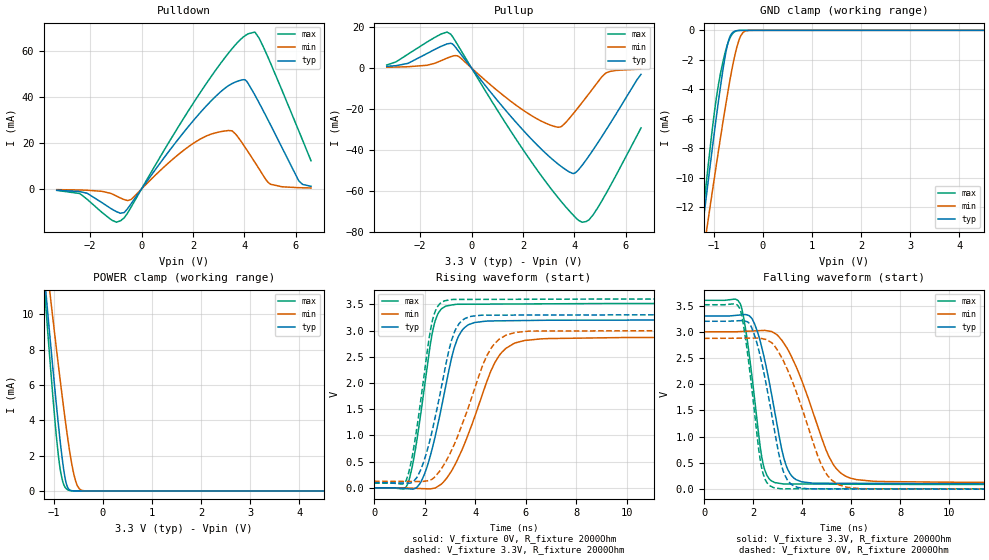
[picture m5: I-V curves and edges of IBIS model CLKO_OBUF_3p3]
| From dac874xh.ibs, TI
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|   CLKO_OBUF_3p3 Model
[Model]   CLKO_OBUF_3p3
Model_type   3-state
Polarity   Non-Inverting
Vmeas = 1.65
Vref = 0
Cref = 2pF
Rref = 100000
|   typ   min   max
C_comp   6.24499E-13   5.18659E-13   6.49121E-13
| Where nom  PVT is Nominal Process, 3.3V, 27C
|   Fast PVT is Strong Process,  3.6V, -40C
|   Slow PVT is Weak Process,   3.0V, 150C
[Voltage Range]   3.3   3   3.6
[Temperature Range]   27   150   -40
[Pullup Reference]   3.3   3   3.6
[Pulldown Reference]   0   -0   0
[Power Clamp Reference]   3.3   3   3.6
[GND Clamp Reference]   0   0   0
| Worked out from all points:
|   slope of the pulldown table from 0 to 0.495 V, typ, clamps not added: 63.8 ohm
|   slope of the pullup table from 0 to 0.495 V, typ, clamps not added: 62.5 ohm
|   GND clamp passes 1 mA (typ) near -0.72 V on its own axis
|   POWER clamp passes 1 mA (typ) near -0.79 V on its own axis
|   falling waveform, V_fixture 3.3V, R_fixture 2000Ohm: 20-80 % time 803ps typ, 1.35ns min, 551ps max; typ from 3.3 V to 0.101 V
|   rising waveform, V_fixture 0V, R_fixture 2000Ohm: 20-80 % time 869ps typ, 1.35ns min, 628ps max; typ from 0 V to 3.2 V
|   rising waveform, V_fixture 3.3V, R_fixture 2000Ohm: 20-80 % time 863ps typ, 1.32ns min, 614ps max; typ from 0.101 V to 3.3 V
|   falling waveform, V_fixture 0V, R_fixture 2000Ohm: 20-80 % time 786ps typ, 1.3ns min, 537ps max; typ from 3.2 V to 0 V
[Pulldown]
|   Voltage   I(typ)   I(min)   I(max)
-3.3V     -518.9uA   -279.8uA   -604.3uA
-2.122V   -1.843mA   -540.5uA   -4.429mA
-815.1mV  -10.56mA   -3.943mA   -13.82mA
-409.2mV  -6.481mA   -4.563mA   -7.949mA
1.591V    23.93mA    16.4mA     29.86mA
2.838V    39.75mA    24.31mA    50.92mA
3.521V    45.83mA    25.31mA    60.97mA
3.957V    47.54mA    19.39mA    66.05mA
4.402V    41.11mA    11.81mA    68.25mA
5.026V    27.83mA    2.052mA    54.68mA
6.125V    3.502mA    572uA      25.23mA
6.6V      1.16mA     444.7uA    12.24mA
[GND Clamp]
|   Voltage   I(typ)   I(min)   I(max)
-3.3V     -72.02mA   -64.29mA   -82.15mA
-1.241V   -13.64mA   -15.69mA   -13.06mA
-1.122V   -10.42mA   -12.98mA   -9.355mA
-993.3mV  -7.012mA   -10.1mA    -5.674mA
-904.2mV  -4.759mA   -8.138mA   -3.641mA
-815.1mV  -2.685mA   -6.23mA    -2.133mA
-726mV    -1.033mA   -4.408mA   -990.6uA
-656.7mV  -325.7uA   -3.092mA   -426.6uA
-577.5mV  -63.94uA   -1.78mA    -100.6uA
-448.8mV  -2.544uA   -357.2uA   -3.784uA
-290.4mV  0A         -7.658uA   0A
6.6V      0A         0A         0A
[Pullup]
|   Voltage   I(typ)   I(min)   I(max)
-3.3V     817.2uA    383.7uA    1.455mA
-2.478V   2.247mA    609.1uA    6.718mA
-815.1mV  12.09mA    5.491mA    16.62mA
-488.4mV  7.958mA    5.563mA    10.23mA
1.591V    -24.53mA   -16.86mA   -32.08mA
3.115V    -44.31mA   -28.13mA   -59.39mA
3.482V    -48.07mA   -28.74mA   -65.15mA
3.947V    -51.62mA   -22.56mA   -71.8mA
4.303V    -47.67mA   -16.95mA   -75.44mA
4.58V     -42.88mA   -12.44mA   -74.2mA
5.234V    -30.43mA   -2.429mA   -61.5mA
6.6V      -3.103mA   -587uA     -29.3mA
[POWER Clamp]
|   Voltage   I(typ)   I(min)   I(max)
-3.3V     80.47mA    68.12mA    94.19mA
-1.191V   12.15mA    13.96mA    11.48mA
-1.112V   9.721mA    12.02mA    8.578mA
-1.082V   8.821mA    11.29mA    7.514mA
-963.6mV  5.325mA    8.441mA    3.54mA
-904.2mV  3.682mA    7.05mA     1.926mA
-854.7mV  2.417mA    5.918mA    969.8uA
-795.3mV  1.132mA    4.602mA    335.3uA
-706.2mV  139.5uA    2.774mA    51.25uA
-557.7mV  1.416uA    575.4uA    830.4nA
-399.3mV  0A         15.59uA    0A
6.6V      0A         0A         0A
[Ramp]
R_load = 2000
|   typ   min   max
dV/dt_r   1.92066/8.65823e-10   1.72468/1.34621e-09   2.10962/6.25538e-10
dV/dt_f   1.91945/7.99727e-10   1.72446/1.34831e-09   2.10598/5.50426e-10
[Falling Waveform]
V_fixture = 3.3V
V_fixture_min = 3V
V_fixture_max = 3.6V
R_fixture = 2000Ohm
C_fixture = 0F
|   Time   V(typ)   V(min)   V(max)
0s        3.3V       3V         3.6V
1.479ns   3.321V     3.005V     3.534V
1.976ns   3.235V     3.016V     2.071V
2.297ns   2.813V     3.023V     792.3mV
2.467ns   2.482V     3.027V     381.2mV
3.213ns   675.6mV    2.813V     101mV
3.759ns   180.9mV    2.334V     98.25mV
5.267ns   112.5mV    474.7mV    95.88mV
6.888ns   109.6mV    151.3mV    93.33mV
125ns     100.9mV    125.9mV    90.03mV
[Rising Waveform]
V_fixture = 0V
V_fixture_min = 0V
V_fixture_max = 0V
R_fixture = 2000Ohm
C_fixture = 0F
|   Time   V(typ)   V(min)   V(max)
0s        959.2pV    17.18nV    795.5pV
1.243ns   -13.82mV   -1.839mV   -2.877mV
1.509ns   -23.58mV   -6.982mV   399.7mV
1.838ns   100.9mV    -13.34mV   1.38V
2.416ns   979.1mV    -2.312mV   3.182V
3.213ns   2.731V     454.6mV    3.499V
3.759ns   3.117V     1.067V     3.502V
4.936ns   3.185V     2.515V     3.505V
6.74ns    3.196V     2.844V     3.509V
125ns     3.201V     2.874V     3.516V
[Rising Waveform]
V_fixture = 3.3V
V_fixture_min = 3V
V_fixture_max = 3.6V
R_fixture = 2000Ohm
C_fixture = 0F
|   Time   V(typ)   V(min)   V(max)
0s        100.9mV    125.9mV    90.03mV
1.207ns   91.03mV    122.6mV    88.89mV
1.458ns   95.42mV    122mV      473.8mV
1.749ns   247mV      121.2mV    1.332V
2.354ns   1.208V     186.9mV    3.274V
3.075ns   2.828V     728.8mV    3.591V
3.563ns   3.22V      1.315V     3.593V
4.631ns   3.293V     2.665V     3.594V
6.209ns   3.295V     2.99V      3.596V
125ns     3.3V       3V         3.6V
[Falling Waveform]
|Gnd
V_fixture = 0V
V_fixture_min = 0V
V_fixture_max = 0V
R_fixture = 2000Ohm
C_fixture = 0F
|   Time   V(typ)   V(min)   V(max)
0s        3.201V     2.874V     3.516V
1.458ns   3.212V     2.878V     3.443V
1.892ns   3.129V     2.88V      2.15V
2.241ns   2.638V     2.878V     725.3mV
2.393ns   2.327V     2.867V     323mV
3.142ns   485.2mV    2.53V      7.241mV
3.621ns   72.53mV    2.031V     7.213mV
4.936ns   5.315mV    331.5mV    7.135mV
6.341ns   3.978mV    10.67mV    7.051mV
125ns     523.1pV    17.17nV    793.6pV
